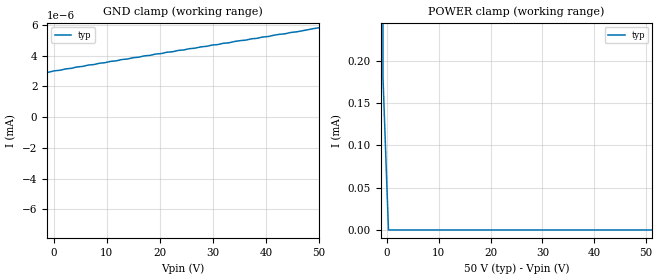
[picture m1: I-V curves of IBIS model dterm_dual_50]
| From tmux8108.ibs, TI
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| dterm_dual_50
[Model]   dterm_dual_50
Model_type   Terminator
|   typ   min   max
C_comp   1.008417e-11   NA   NA
[Voltage Range]   50   NA   NA
[Temperature Range]   27   NA   NA
[Power Clamp Reference]   50   NA   NA
[GND Clamp Reference]   0   NA   NA
[GND Clamp]
|   Voltage   I(typ)   I(min)   I(max)
-55V      -4.512A    NA         NA
-50.76V   -2.368mA   NA         NA
-49.7V    -674.8pA   NA         NA
-44.39V   -345.7pA   NA         NA
-34.85V   541.4pA    NA         NA
-26.36V   1.244nA    NA         NA
-13.64V   2.149nA    NA         NA
6.515V    3.384nA    NA         NA
50V       5.811nA    NA         NA
[POWER Clamp]
|   Voltage   I(typ)   I(min)   I(max)
-5V       1.488A     NA         NA
-1.818V   290.8mA    NA         NA
-757.6mV  181uA      NA         NA
303mV     5.798nA    NA         NA
100V      -717.1pA   NA         NA
